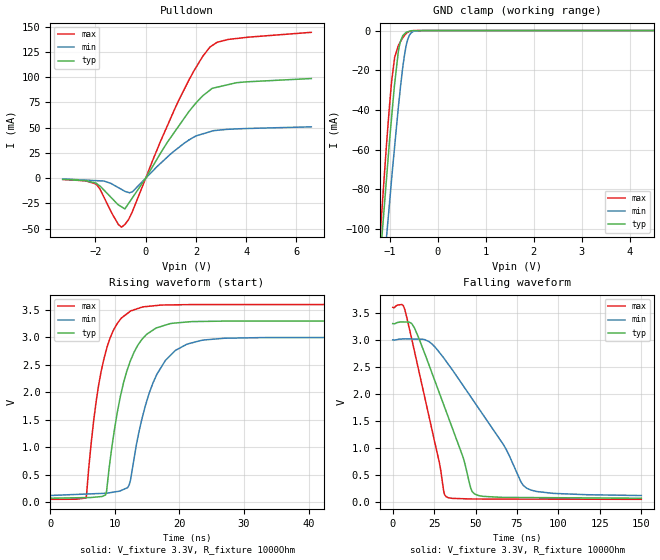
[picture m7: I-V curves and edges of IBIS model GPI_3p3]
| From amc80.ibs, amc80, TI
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|   GPI model
[Model]  GPI_3p3
Model_type   I/O_open_drain
Polarity   Non-Inverting
Enable   Active-Low
Vinl = 0.8
Vinh = 2
Vmeas = 1.65
Vref = 1.65
Cref = 15pF
Rref = 50
|   typ   min   max
|   (nom PVT)   (Fast PVT)   (slow PVT)
|   BUFFER OUTPUT TURNED HIGH or as in INPUS
|C_comp   9.696E-13   9.122E-13   1.014E-12
|   BUFFER OUTPUT TURNED LOW
C_comp   9.122E-13   8.955E-13   1.092E-12
| Where   nom PVT is  Nominal Process, 3.3V, 27C
|   Fast PVT is Strong Process, 3.6V, -40C
|   Slow PVT is Weak Process, 3.0V, 125C
|C_comp - from L-C Tank method, L = 1nH, peak frequency
[Voltage Range]   3.3   3   3.6
[Temperature Range]   27   125   -40
[Pullup Reference]   3.3   3   3.6
[Pulldown Reference]   0   0   0
[Power Clamp Reference]   3.3   3   3.6
[GND Clamp Reference]   0   0   0
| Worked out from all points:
|   slope of the pulldown table from 0 to 0.495 V, typ, clamps not added: 23.9 ohm
|   GND clamp passes 1 mA (typ) near -0.66 V on its own axis
|   falling waveform, V_fixture 3.3V, R_fixture 1000Ohm: 20-80 % time 23ns typ, 36.2ns min, 15.5ns max; typ from 3.3 V to 0.076 V
|   rising waveform, V_fixture 3.3V, R_fixture 1000Ohm: 20-80 % time 3.47ns typ, 4.16ns min, 2.9ns max; typ from 0.076 V to 3.3 V
[Pulldown]
|   Voltage   I(typ)   I(min)   I(max)
-3.3V     -1.175mA   -709.3uA   -1.236mA
-1.968V   -5.008mA   -2.409mA   -5.947mA
-1.088V   -26.36mA   -9.306mA   -45.71mA
-962mV    -28.32mA   -11.08mA   -48.44mA
-827.4mV  -30.42mA   -12.97mA   -45.84mA
-525mV    -19.31mA   -13.41mA   -32.78mA
593.7mV   24.85mA    14.71mA    36.61mA
1.332V    52.15mA    30.66mA    77.79mA
1.893V    71.19mA    40.3mA     105mA
2.561V    87.17mA    45.99mA    129.8mA
3.291V    92.6mA     48.36mA    137.3mA
6.59V     98.58mA    50.8mA     144.3mA
[GND Clamp]
|   Voltage   I(typ)   I(min)   I(max)
-3.3V     -813.1mA   -775.3mA   -896.6mA
-1.228V   -123.5mA   -149.7mA   -112mA
-1.173V   -106.1mA   -133.8mA   -93.1mA
-1.072V   -75.26mA   -104.8mA   -58.01mA
-971mV    -45.77mA   -76.94mA   -27.69mA
-900.7mV  -26.96mA   -58.47mA   -13.55mA
-827.4mV  -11.32mA   -39.73mA   -7.849mA
-784.4mV  -5.869mA   -29.71mA   -5.837mA
-659.3mV  -890.4uA   -7.474mA   -1.463mA
-554.2mV  -121.2uA   -1.098mA   -245.8uA
-324.6mV  -54.66uA   -2.897uA   -5.777uA
6.59V     0A         0A         0A
[POWER Clamp]
|   SCR cell for ESD function. Effects occurr above VDD x 2
|   Voltage   I(typ)   I(min)   I(max)
-3.3V     0A         0A         0A
0V        0A         0A         0A
6.6V      0A         0A         0A
[Ramp]
R_load = 1000
|   typ   min   max
dV/dt_r   1.93427/3.46653e-009   1.7245/4.10749e-009   2.12651/2.90242e-009
dV/dt_f   1.93427/2.30234e-008   1.7245/3.62212e-008   2.12651/1.55455e-008
[Falling Waveform]
V_fixture = 3.3V
V_fixture_min = 3V
V_fixture_max = 3.6V
R_fixture = 1000Ohm
C_fixture = 0F
|   Time   V(typ)   V(min)   V(max)
0s        3.3V       3V         3.6V
7.287ns   3.33V      3.019V     3.56V
13.39ns   3.202V     3.014V     2.753V
21.85ns   2.54V      2.969V     1.593V
30.93ns   1.789V     2.66V      182.3mV
32.23ns   1.681V     2.605V     105.6mV
42.24ns   850.2mV    2.167V     67.22mV
47.98ns   197.7mV    1.909V     62.03mV
80.51ns   88.8mV     268.2mV    60.05mV
150ns     76.22mV    125.8mV    55.81mV
[Rising Waveform]
V_fixture = 3.3V
V_fixture_min = 3V
V_fixture_max = 3.6V
R_fixture = 1000Ohm
C_fixture = 0F
|   Time   V(typ)   V(min)   V(max)
0s        76.22mV    125.8mV    55.81mV
5.537ns   87.41mV    151.9mV    81.51mV
7.083ns   97.35mV    159.1mV    1.816V
8.577ns   137.9mV    166.1mV    2.73V
10.42ns   1.667V     198.7mV    3.263V
12.23ns   2.514V     319.1mV    3.463V
14.29ns   2.977V     1.562V     3.555V
17.83ns   3.225V     2.582V     3.591V
23.81ns   3.292V     2.955V     3.599V
150ns     3.3V       3V         3.6V
